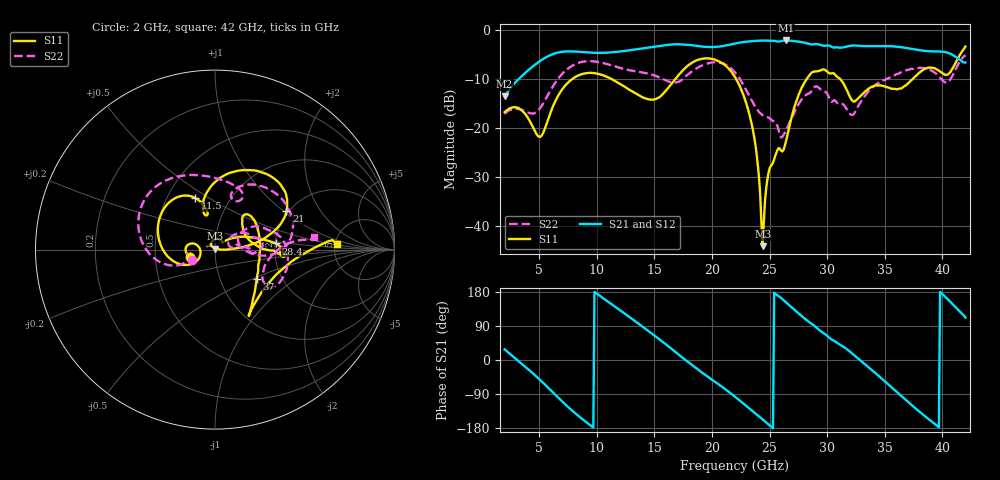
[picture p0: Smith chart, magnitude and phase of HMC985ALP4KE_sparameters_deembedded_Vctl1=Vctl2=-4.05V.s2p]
!s2p File: Measurements: S11, S21, S12, S22
# GHz S dB R 50.0
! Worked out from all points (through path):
!   401 points, 2 GHz to 42 GHz, reference 50 ohm
!   highest |S21| = -2.11 dB at 26.4 GHz (marker M1); lowest = -13.5 dB at 2 GHz (marker M2)
!   lowest |S11| = -44.0 dB at 24.4 GHz (marker M3), VSWR 1.01, Z = 50.2 + j0.612 ohm
!   |S11| at or under -10 dB: start of sweep to 7.852 GHz; 22.1 GHz to 28.21 GHz (6.11 GHz wide, 24.3 % of centre); 31.14 GHz to 37.4 GHz (6.265 GHz wide, 18.3 % of centre)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
!   |S22| runs from -21.9 to -5.1 dB; largest |S21 - S12| = 0.00065
!   S11 on the Smith chart (normalised r, x): 2 GHz: 0.75, -0.07; 11.5 GHz: 0.69, +0.44; 21 GHz: 1.95, +1.04; 28.4 GHz: 2.01, +0.16; 37 GHz: 1.49, -0.53; 42 GHz: 5.17, +0.58
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2  -16.72 -162.7  -13.49 28.2  -13.49 28.2  -17.05 -156.7
5.1  -21.74 -170.0  -6.26 -53.1  -6.26 -53.1  -15.85 -159.7
6.3  -14.98 -151.4  -4.80 -88.6  -4.80 -88.6  -11.05 -162.4
8.7  -8.97 149.8  -4.47 -154.9  -4.47 -154.9  -6.49 150.7
11.5  -10.25 110.8  -4.49 142.6  -4.49 142.6  -7.35 104.5
13.6  -13.21 101.6  -3.86 96.4  -3.86 96.4  -8.48 75.2
15.4  -13.72 106.7  -3.26 55.5  -3.26 55.4  -9.62 62.2
17.9  -7.25 79.3  -2.99 -4.8  -2.99 -4.8  -9.07 71.8
21  -6.91 28.2  -3.22 -73.4  -3.23 -73.4  -6.83 17.0
22  -9.56 16.5  -2.74 -97.0  -2.74 -96.9  -8.62 -0.2
23.5  -19.69 2.9  -2.24 -134.3  -2.24 -134.3  -14.54 -4.6
24.4  -44.01 75.5  -2.13 -157.0  -2.13 -157.0  -17.33 8.6
25  -28.18 126.4  -2.16 -172.3  -2.16 -172.3  -17.95 12.2
26.4  -22.90 41.5  -2.11 152.9  -2.11 152.9  -20.51 33.9
28.4  -9.37 5.8  -2.79 100.8  -2.79 100.8  -12.91 17.4
28.7  -8.58 0.8  -2.92 94.6  -2.93 94.6  -12.19 15.6
32.4  -14.53 30.7  -3.14 11.1  -3.14 11.0  -16.79 26.8
33.9  -11.51 47.7  -3.26 -27.0  -3.27 -27.1  -11.71 30.1
35.4  -11.76 17.3  -3.27 -67.1  -3.27 -67.0  -9.72 18.5
37  -10.91 -35.3  -3.69 -110.2  -3.69 -110.2  -8.09 3.8
39.8  -8.44 -55.7  -4.37 179.6  -4.37 179.6  -9.68 -34.1
42  -3.36 2.6  -6.60 112.1  -6.61 112.1  -5.10 7.5
